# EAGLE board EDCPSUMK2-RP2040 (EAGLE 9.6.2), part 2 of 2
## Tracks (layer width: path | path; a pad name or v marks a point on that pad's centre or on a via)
1V1MCU  (via drill 0.3, 0.4)
  Top 0.203: U1.23 81.57,40.41 81.06,39.9 v81.06,39.74 | U1.45 88.21,39.21 87.54,39.88 87.54,41.22 v87.83,41.51 88.13,41.21 U1.50
  Bottom 0.203: C32.2 79.91,39.12 80.86,39.12 81.06,39.32 v81.06,39.74 82.73,39.74 83.25,39.22 87.47,39.22 87.5,39.25 | v87.83,41.51 87.54,41.22 87.54,39.29 87.5,39.25 | 87.5,39.25 87.5,38.11 C46.1 87.58,38.03 87.58,36.08 C33.2
3V3MCU  (via drill 0.3, 0.35, 0.4, 0.4 pad 0.9, 0.41 pad 0.81, 0.41 pad 0.91)
  Top 0.203: 39.17,32.42 39.17,34.39 C60.2 v40.17,36.38 | v80.92,40.6 81.13,40.81 U1.22 | R53.2 75.84,34.32 v75.19,34.32 | v91.78,36.41 91.29,36.91 91.29,38.01 90.49,38.81 U1.44 87.85,38.81 | U1.33 84.62,38.88 84.84,39.1 87.56,39.1 87.85,38.81 | 87.85,38.81 88.22,38.44 U1.42 88.22,35.7 89.01,34.91 C7.2 | U1.10 84.62,43.09 84.77,42.94 87.95,42.94 | 87.95,42.94 87.96,42.94 88.23,43.2 U1.1 | v87.96,43.38 87.96,42.95 87.95,42.94 | U1.49 88.26,40.81 88.1,40.65 v88.1,40.57 88.26,40.41 U1.48
  Top 0.305: J6.2 42.07,58.84 C25.2 | 41.83,52.58 C26.1 41.89,52.79 39.93,50.83 D3.2 | 2.28,36.83 R13.2 | U6.14 63.22,43.16 63.22,43.28 63.12,43.38 v62.4,43.38 65.71,46.69 C52.2 66.25,48.27 R15.1 | U3.14 70.06,40.65 69.92,40.51 v69.74,40.51 | U9.1 11.6,10.54 11.3,10.24 v11.02,10.24 v11.02,10.25 | R52.2 78.58,16 79.58,17.01 80.02,17.01 v80.3,17.29 | v14.29,19.85 14.29,21.84 K1.4 14.34,23.2 14.35,23.2 14.35,25.1 13.4,26.05 12.82,26.05 12.48,26.38 | 12.48,26.38 D7.2 | C57.1 9.45,25.95 10.12,25.95 | 10.12,25.95 12.05,25.95 12.48,26.38 | v10.07,26 10.12,25.95 | v46.01,40.72 47.28,41.99 48.53,41.99 LS1.1 | U2.3 39.01,32.26 39.17,32.42 | U5.8 78.31,57.28 v76.88,57.28
  Top 0.61: C25.2 41.83,52.58 | 2.28,36.83 C2.2 | R54.2 90.49,15.33 v89.82,16.01 | R35.1 58.67,49.62 58.32,49.28 v58.32,48.77 | R66.1 56.53,49.27 v56.29,49.03 | C44.2 28.08,33.71 v27.6,34.19 27.4,34.39 U7.1 | C7.2 90.9,34.91 C16.2 C45.1 92.37,35.78 | 92.39,35.8 92.37,35.78 | 92.37,35.78 92.37,35.83 v91.78,36.41
  Top 0.813: R13.2 1.63,36.87 v0.92,37.58
  PWR 0.305: v14.29,19.85 14.29,17.82 10.46,13.99 10.46,10.8 v11.02,10.25 | v0.92,37.58 0.92,35.51 | v10.07,26 8.75,26 8.04,26.71 8.04,28.91 7.83,29.12 3.6,29.12 2.59,30.13
  Bottom 0.203: v80.92,40.6 80.89,40.57 79.89,40.57 C50.2 | R40.2 78.17,55.88 v77.07,54.78
  Bottom 0.305: C20.2 61.25,43.06 62.08,43.06 v62.4,43.38 | v40.17,36.38 39.23,37.32 C51.2 | v91.78,36.41 91.8,36.41 92.55,35.66 R57.2 | 3V3MCU.TP 77.83,54.02 v77.07,54.78 | v76.88,57.28 78.66,59.06 81.7,59.06 C8.2 81.72,57.58 C15.1
  Bottom 0.61: D2.2 21.9,34.64 23.06,33.49 26.89,33.49 v27.6,34.19 | C53.2 v69.75,40.52 v69.74,40.51 | v89.82,16.01 89.86,16.05 89.86,18.4 90.5,19.04 90.5,21.93 90.36,22.07 | R19.2 90.36,22.07 | v87.96,43.38 87.45,43.89 | 87.45,43.89 C5.2 C6.2 | JP1.1 94.4,42.88 v94.4,43.49 | C31.2 87.45,43.89 | C12.2 88.01,25.69 88.01,24.45 88.69,23.77 89.41,23.77 90.5,22.68 90.5,22.21 90.36,22.07
  other vias: 72.48,54.67 73.17,55.87 74.11,56.29 73.17,56.91 73.13,57.69 73.1,58.55 74.09,57.38 75.07,54.8 76.81,56.25
  pour PWR (isolate 0.305, rank 3): -0.25,28.74 -0.25,53.44 7.21,60.9 91.95,60.9 97.18,55.67 97.18,7.88 74.15,7.88 74.15,50.26 70.2,50.26 70.2,36.19 35.77,35.9 32.88,32.99 11.08,33.28 11.08,49.14 4.17,49.14 3.97,28.74
  pour Top: 70.1,60.33 72.91,60.33 74.92,58.32 76.94,58.32 77.33,57.93 77.33,54.11 77.36,54.08 71.82,54.08 70.1,55.8
3V_REF  (via drill 0.35)
  Top 0.203: U1.43 90.25,38.41 90.77,37.89 90.77,37.04 89.59,35.86 v89.08,35.86
  Bottom 0.305: R57.1 89.62,32.35 89.39,32.12 | 89.39,32.12 89.39,29.32 90,28.71 C66.2 91.23,28.5 U8.1 | v89.08,35.86 89.06,35.86 89.06,32.45 89.39,32.12
BUZZ  (via drill 0.3)
  Top 0.203: U1.32 84.24,37.55 84.24,36.16 v84.29,36.11
  Bottom 0.305: R28.1 67.12,39.28 75.56,39.28 79.79,35.05 83.84,35.05 84.29,35.5 v84.29,36.11
CC1
  Bottom 0.305: J1.3 18.44,7.11 16.55,9 16.55,12.05 15.38,13.23 U10.13 10.91,13.23 9.51,14.62 7.82,14.62 R55.2
CC2
  Bottom 0.305: J1.9 15.45,7.65 15.45,11.85 14.72,12.57 U10.12 8.02,12.57 R56.2
CS
  Top 0.305: J6.7
  Top 0.61: J6.7 R29.2 R66.2
D0
  Top 0.305: J6.3
  Top 0.61: R14.2 J6.3
D1
  Top 0.305: J6.4
  Top 0.61: R17.2 J6.4
DSP_RST  (via drill 0.3, 0.3 pad 0.64)
  Top 0.203: U1.9 85.02,45.85 v84.19,46.68
  Top 0.305: R21.1 49.7,51.92 49.7,49.08 v49.68,49.05
  Bottom 0.203: v84.19,46.68 84.06,46.81 79.37,46.81 78.69,46.12 72.97,46.12 72.26,45.41 72.26,43.98 71.65,43.37 70.53,43.37 68.16,45.75 53.07,45.75 49.72,49.09 v49.68,49.05
EN_DCDC  (via drill 0.3, 0.3 pad 0.64)
  Top 0.203: U1.4 87.02,46.16 v87.42,46.56 v87.42,46.57
  Top 0.305: R31.1 61.57,48.57 v61.62,48.52
  Bottom 0.203: v87.42,46.57 86.32,46.57 85.14,47.76 78.74,47.76 78.04,47.06 69.84,47.06 69.42,47.48 62.93,47.48 62.43,46.98 60.09,46.98
  Bottom 0.305: v61.62,48.52 60.09,46.98 59.58,46.48 53.73,46.48 50.39,49.81 33.85,49.81 33.15,49.11 22.64,49.11 16.03,42.5 13.66,42.5 12.8,43.35 12.8,44.44 11.93,45.31 11.93,48.62 R27.2
EN_TPS54531  (via drill 0.3 pad 0.64)
  Top 0.305: U12.3 10.05,46.02 v9.8,46.28
  Bottom 0.305: 8.14,41.45 7.52,40.84 Q4.2 | v9.8,46.28 8.15,44.63 8.15,41.46 8.14,41.45 | 8.14,41.45 R43.2 6.08,39.76 5.41,39.09 EN_TPS54531.TP
FB
  Top 0.203: U11.1 70.05,47.99 70.28,47.76 FB_ADJ.2
FB_DAC
  Top 0.305: R30.1 36.7,34.16 U2.1
GND  (via drill 0.3, 0.3 pad 0.6, 0.3 pad 0.64, 0.35, 0.4, 0.4 pad 0.9, 0.41, 0.41 pad 0.81, 0.41 pad 0.91, 1.5 pad 2.5)
  Top 0.203: U1.19 84.17,42.01 v84.4,42.24 | 90.9,33.11 C16.1 | U2.2 v37.9,33.01 | U1.57 85.61,41.02 v85.61,41.08 | U12.9 14,46.76 v14,46.99
  Top 0.305: 19.33,47.4 C38.1 | U6.7 57.42,38.73 v56.79,38.1 | U7.9 18.31,30.65 v17.7,30.65 17.22,30.65 R50.2 14.63,33.24 C58.1 | Q5.2 5.52,15.93 R49.1 6.7,19.02 v8.32,20.65 8.32,21.72 C57.2 | C54.1 69.61,45.09 v70.84,45.09 | v62.74,34.65 64.45,34.65 65.56,33.54 C48.1 | C2.1 4.18,34.68 6.75,34.68 v6.76,34.67 6.55,34.67 5.87,35.36 S2.2 | v12.31,30.27 12.81,29.77 D7.1 | v41.99,36.48 41.99,35.41 C60.1 41.97,34.64 41.5,34.17 U2.6 | R16.2 64.66,50.11 Q2.2 | v74.19,59.83 74.46,59.56 DZ1.2 76.18,59.56 v76.41,59.79 | 1.93,41.78 1.71,41.56 | U12.7 15.47,47.3 v15.01,47.76 | C65.1 32.34,31.61 32.99,31.61 v33.06,31.68 33.8,31.68 R45.1 | C27.1 49.92,33.48 v50.25,33.81 | U3.7 73.95,37.35 75.04,38.44 C61.1 75.24,38.47 75.24,39.95 75.55,40.26 X1.2 76.2,40.31 v76.2,41.68 | U4.2 U4.1 39.02,39.88 v38.49,39.35 | 78.67,45.16 78.67,44.17 X1.4 | 78.67,45.16 C59.1 | U5.4 83.45,50.3 v83.48,50.27 | v79,45.49 78.67,45.16 | C16.1 91.64,32.37 v91.64,31.15
  Top 0.508: 1.68,45.79 1.71,45.76 C21.2 1.64,44.67 0.57,44.67 | 4.62,45.6 4.6,45.58 C17.2 4.6,43.79 | C18.2 7.55,44.52 7.55,45.65 | 4.6,43.79 | C18.2 7.56,43.76 7.54,43.74 | C18.2 7.57,44.52 8.82,44.52
  Top 0.61: 19.33,47.4 19.33,47.88 19.64,48.19 R44.1 19.64,50.44 v19.7,50.51 | v23.55,45.35 22.84,44.64 C34.1 | v95.02,16.06 94.44,16.65 C24.1 | U7.9 U7.10 | v18.44,34.17 18.51,34.23 U7.8 U7.7 | C44.1 27.77,31.91 27.66,31.8 v27.46,31.8 27.4,31.74 U7.16 | C26.2 40.03,52.79 C25.1 40.03,55.94 J6.1 | C11.1 55.19,37.86 56.55,37.86 v56.79,38.1 | C49.1 67.05,40.76 66.49,40.2 v66.38,40.2 | C47.1 v70.84,45.09 | v54.38,47.25 54.94,47.25 C9.2 | Q2.2 64.63,48.85 v64.62,48.82 | R18.1 59.65,42.36 v59.33,42.04 | 85.46,9.49 v85.3,9.33 | v62.74,34.65 62.7,34.69 C14.1 | 18.35,23.28 K1.9 18.35,22.12 18.46,22.23 v19.04,22.23 | 18.35,23.28 18.35,23.51 18.33,23.51 18.33,26.67 v18.3,26.71 17.35,25.75 K1.8 | C45.2 C16.1 90.9,33.11 | C16.1 89.47,33.09 C7.1 | v19.29,23.28 18.35,23.28 | v19.3,21.02 18.41,21.02 18.35,20.96
  Top 0.813: C21.2 1.71,41.56 v0.79,40.64 | OP1.3 85.46,9.49 | C10.1 1.93,41.78 | v19.55,15.3 19.81,15.04 RSENSE.2
  Top 1.016: R59.1 17.6,15.3 v19.55,15.3 | D6.1 13,54.63 | D6.1 15.33,51.7 | D6.1 15.33,57.6 | D6.1 15.65,54.3 17.15,54.3
  Top 1.27: C21.2 4.57,44.6 C17.2 7.44,44.63 C18.2
  Bottom 0.203: 85.45,45.64 86.76,45.64 C5.1 v87.62,45.71 C31.1
  Bottom 0.305: v18.44,34.17 18.92,34.64 D2.1 | v12.31,30.27 12.31,29.05 C35.2 | C36.1 6.76,32.67 v6.76,34.67 | D8.2 14.46,39.94 12.69,41.71 v9.04,41.71 | C28.1 5.95,45.19 5.95,44.68 6.28,44.35 6.28,44.05 6.4,44.05 v6.5,43.95 | v9.04,41.71 9.16,41.83 9.16,43.67 C30.1 | R43.1 9.94,40.81 v9.04,41.71 | C15.2 83.55,59.05 C8.1 v84.58,59.08 v84.59,59.09 | C51.1 37.86,34.42 37.91,34.37 v37.91,33.02 v37.9,33.01 | C12.1 89.98,25.83 | Q9.2 60.86,35.83 R32.2 62.05,35.34 v62.74,34.65 | C32.1 78.11,39.16 C50.1 77.29,40.59 v76.2,41.68 | C42.2 23.71,45.51 v23.55,45.35 | U8.2 92.7,30.51 C66.1 91.64,31.13 v91.64,31.15 | GND.TP 40.42,58.5 39.53,57.61 J6.1
  Bottom 0.61: 31.69,45.59 C39.2 31.63,45.53 35.91,45.53 36.2,45.81 v36.2,46.66 | C53.1 72.55,40.21 72.72,40.04 v72.81,40.04 | C22.1 82.82,20.19 v82.96,20.32 | C23.1 80.66,23.49 v80.55,23.37 | C20.1 60.11,41.27 v59.33,42.04 | S1.SW- 89.98,25.66 89.98,25.83 | C6.1 85.45,45.64 | 86.58,45.64 86.78,45.66 C5.1 | JP1.3 JP1.5 JP1.7 JP1.9 94.02,36.21 v94.06,36.17 | C46.2 85.83,37.98 C33.1 85.19,36.03 v85.12,36.09
  Bottom 0.813: C42.2 C40.2 28.61,45.56 31.56,45.56 C39.2 | R22.2 82.28,12.17 v82.66,11.79
  Bottom 1.016: v20.92,22.07 20.92,23.74 20.5,24.16
  other vias: 13.54,53.09 14.25,47.76 13.49,47.76 13.23,46.99 14.76,46.99 15.01,46.23 14.25,46.23 13.49,46.23 13.23,45.47 14,45.47 14.76,45.47 14.27,50.96 14.77,51.96 15.27,50.96 16.27,50.96 15.77,51.96 16.77,51.96 17.27,50.96 17.77,51.96 17.27,52.96 13.77,51.96 9.77,56.46 10.77,56.46 11.77,56.46 12.77,56.46 20.77,50.96 13.77,56.46 21.77,50.96 22.77,50.96 11.32,59.76 12.32,59.76 13.32,59.76 14.32,59.76 15.32,59.76 16.32,59.76 17.32,59.76 18.32,59.76 19.32,59.76 20.32,59.76 21.32,59.76 22.32,59.76 23.32,59.76 24.32,59.76 25.32,59.76 26.32,59.76 27.32,59.76 15.82,50.26 10.82,58.76 11.82,58.76 12.82,58.76 13.82,58.76 14.82,58.76 15.82,58.76 16.82,58.76 17.82,58.76 18.82,58.76 19.82,58.76 20.82,58.76 21.82,58.76 22.82,58.76 23.82,58.76 24.82,58.76 25.82,58.76 26.82,58.76 14.82,50.26 11.32,57.76 12.32,57.76 13.32,57.76 14.32,57.76 15.32,57.76 16.32,57.76 17.32,57.76 18.32,57.76 19.32,57.76 20.32,57.76 21.32,57.76 22.32,57.76 23.32,57.76 24.32,57.76 25.32,57.76 26.32,57.76 9.4,55.3 10.4,55.3 11.4,55.3 12.4,55.3 9.9,54.3 10.9,54.3 11.9,54.3 12.9,54.3 9.4,53.3 10.4,53.3 11.4,53.3 12.4,53.3 9.9,52.3 10.9,52.3 11.9,52.3 12.9,52.3 28.97,51.23 29.99,51.23 31.11,51.27 32.21,51.31 6.5,44.69 18.95,16.5 20.55,16.49 20.92,15.25 72.96,52.92 72.95,51.91 74.2,52.18 75.15,52.17 76.28,52.17 77.14,52.9 77.2,51.7 85.6,42.24 86.81,42.24 86.81,41.08 86.81,39.92 85.6,39.92 84.4,39.92 84.4,41.08 18.27,25.73 19.31,24.43
  pour Bottom: 11.94,49.38 11.94,45.32 12.8,44.45 12.8,43.18 13.57,42.42 15.88,42.42 18.34,44.89 18.34,47.96 18.75,48.37 18.75,49.08 18.44,49.38
  pour Top (no thermals): 85.96,10.47 85.96,8.44 89.77,8.44 89.77,10.47
  pour Top: 8.9,60.3 8.9,52.32 11.42,49.8 33.4,49.8 32.9,50.3 32.9,59.8 32.4,60.3
  pour Bottom (isolate 0.305): 8.41,60.3 8.41,48.79 12.9,44.3 18.4,44.3 22.9,48.8 32.9,48.8 33.4,49.3 33.4,59.8 32.9,60.3
  pour GND (isolate 0.35): -1.04,13.55 24.58,13.55 24.58,27.1 74.2,27.1 74.2,5 97.89,5 97.89,54.02 89.91,62 6.05,62 -1.04,54.91
  pour Top: 18.29,14.04 21.73,14.04 21.73,17.59 18.29,17.59
  pour Top: 0.25,46.26 0.25,43.56 9.22,43.56 9.22,46.34 0.25,46.34 0.25,46.27
  pour Bottom (isolate 0.254): 17.09,28.7 18.78,28.7 18.78,23.84 22.21,23.84 22.21,20.52 16.99,20.52 16.99,28.51
  pour Top: 71.68,53.57 77.4,53.57 77.4,51.38 76.87,50.85 73.36,50.85 72.37,51.84 71.68,51.84
  pour Bottom: 23.44,47.1 36.78,47.1 36.78,44.88 36.48,44.58 22.71,44.58 22.71,46.37
  pour Bottom (isolate 0.254): 22.39,20.57 22.39,28.01 41.36,28.01 41.36,32.72 40.92,33.16 17.77,33.16 16.91,32.3 16.91,20.51
  pour Top (isolate 0.254): 17.4,27.46 19.13,27.46 19.82,26.77 19.82,24.1 20.12,23.8 21.93,23.8 22.39,23.34 22.39,21.33 21.63,20.57 18.98,20.57 18.89,20.66 18.89,23.76 18.39,24.26 17.14,24.26 17.02,24.38 17.02,27.08
GND_IN  (via drill 0.3 pad 0.6, 0.3 pad 0.64, 0.4 pad 0.8)
  Top 0.203: J1.S5 20.19,1.12 D4.3 13.21,1.12 J1.S6
  Top 0.305: R34.1 10.2,16.2 v9.85,16.55 | U9.3 13.55,11.09 13.55,9.45 13.27,9.73 12.55,9.73 U9.2 U9.3
  Top 1.016: C56.2 16.78,7.99 16.78,8.16 16.84,8.11 16.84,9.55 16.63,9.75 C55.2 16.75,11.01 19.56,11.01 RSENSE.1 19.81,8.9 v20.04,8.67
  Bottom 0.203: 6.15,15.55 6.1,15.5 R55.1 5.3,14.6
  Bottom 0.305: 5.3,14.6 4.56,13.86 v4.56,12.68 4.58,12.66 6.09,12.66 R56.1 | J1.12 v13.59,7.62 | J1.1 19.8,7.12 v20.09,7.42 | U10.5 18.11,12.56 18.99,12.56 20.04,11.51 v20.04,8.67 | 6.15,15.55 7.33,16.73 9.67,16.73 v9.85,16.55 5.55,16.55 GND_IN.TP
  other vias: 21.29,8.62 21.29,7.47 12.39,8.67 13.59,8.67 12.44,7.62
  pour GND: -1.3,12.8 24.2,12.8 24.2,-2 -1.3,-2
  pour Top: 7.26,6.8 21.7,6.8 21.7,11.55 7.26,11.55
  pour Bottom (isolate 0.254): 19.4,9.22 22,9.22 22,0.35 11.4,0.35 11.37,0.38 11.37,9.12 11.45,9.2 14.2,9.2 14.2,6.9 13.65,6.9 13.65,2.9 19.5,2.9 19.85,3.25 19.85,5.35 19.4,5.8
IN+  (via drill 0.3 pad 0.6, 0.3 pad 0.64, 0.35, 1.5 pad 2.5)
  Top 0.203: PTC1.2 2.84,29.71
  Top 0.305: 3.32,11.45 3.04,11.73 v2.99,11.73
  Top 0.406: D1.C 2.52,10.18 2.4,10.3
  Top 1.016: C56.1 16.8,6.11 | 16.78,5.03 16.78,6.15 C56.1 | C56.1 16.92,6.05 | v6.4,27.09 5.47,27.09 2.84,29.71
  Bottom 0.305: J1.2 19.05,5.54 18.45,4.94 v18.44,4.94 | R47.1 v21.39,11.05 | v15.03,4.86 14.35,5.54 J1.11 | R62.2 6.07,10.52 4.2,10.52 v2.99,11.73 2.02,12.7 IN+.TP
  Bottom 0.61: R51.1 6.02,36.41 5.08,35.47 C36.2 5.08,30.37 6.43,29.02 6.43,27.12 v6.4,27.09
  other vias: 14.44,3.97 19.06,3.85 16.8,3.9 2.95,10.99 3,9.58
  pour Bottom (isolate 0.254, rank 2): 13.89,5.89 13.89,3.26 19.79,3.26 19.79,5.89
  pour Top: 13.77,6.06 19.79,6.06 19.79,3.29 13.77,3.29
  pour PWR (isolate 0.254): -0.6,28.87 -0.6,10.35 11.05,-1.3 23.9,-1.3 23.9,17.7 23.8,17.8 7.88,17.8 7.88,28.87
  pour Top (isolate 0.305): 2.61,11.99 2.16,11.54 2.16,9.11 3.34,7.93 4.16,7.93 4.46,8.23 4.46,11.59 4.05,12 2.63,12
IN_OVC  (via drill 0.3, 0.35)
  Top 0.305: R48.2 6.7,12.69 R49.2 | R49.2 6.57,14.11 Q5.1 | v12.66,25.19 11,25.19 10.15,24.34 10.15,18.98 8.12,16.95 8.12,14.67 7.63,14.18 R49.2 | v66.46,32.13 66.5,32.17 66.5,39.17 67.21,39.88 68.87,39.88 68.92,39.93 68.92,41.51 69.42,42 70.42,42 70.6,42.18 70.6,43.62 70.35,43.87 64.55,43.87 64.27,43.59 64.27,42.6 64.12,42.45 U6.13
  GND 0.305: v37.06,31.59 36.42,30.94 18.7,30.94 18.25,31.39 16.89,31.39 16.23,30.73 v16.23,30.01
  PWR 0.305: v66.46,32.13 66.3,31.97 40.08,31.97 39.74,32.31 38.98,32.31 38.26,31.59 v37.06,31.59 | v16.23,30.01 15.44,30.01 12.66,27.23 v12.66,25.19
ISENSE  (via drill 0.3, 0.4)
  Top 0.203: U1.39 87.04,37.55 87.04,33.97 86.81,33.74 v86.81,33.59
  Top 0.305: U4.3 41.06,40.84 v40.89,41.02
  Bottom 0.305: v86.81,33.59 86.71,33.49 78.4,33.49 76.16,35.73 73.99,35.73 71.91,37.81 69.11,37.81 65.06,33.76 59.22,33.76 57.57,35.41 45.12,35.41 40.89,39.64 v40.89,41.02 40.47,41.44 ISENSE.TP
MISO  (via drill 0.3, 0.3 pad 0.64)
  Top 0.203: v81.45,36.96 81.23,37.18 81.23,38.49 81.55,38.81 U1.27
  Top 0.305: R24.1 53.12,51.94 v53.49,51.57
  PWR 0.203: v81.45,36.96 81.23,37.18 81.23,37.94 81.46,38.17 87.48,38.17 88.74,39.43 88.74,47.28 88.2,47.82 v87.92,47.82
  Bottom 0.305: v53.49,51.57 53.64,51.42 70.71,51.42 71.57,50.56 82.84,50.56 83.21,50.93 84.26,50.93 87.37,47.82 v87.92,47.82
MOSI  (via drill 0.3, 0.3 pad 0.64)
  Top 0.203: U1.30 83.44,37.55 v83.44,36.25 v83.43,36.24
  Top 0.305: R17.1 48.3,51.94 v48.41,51.82
  PWR 0.203: v83.43,36.24 83.43,36.73 88.33,36.73 90.15,38.56 90.15,47.85 87.3,50.7 v85.37,50.7
  Bottom 0.203: v85.37,50.7 84.63,51.44 84.52,51.44
  Bottom 0.305: v48.41,51.82 50.16,53.57 69.58,53.57 72.06,51.09 77.45,51.09 77.8,51.44 84.52,51.44
N$1
  Top 0.305: U7.6 21.05,36.9 21.72,37.57 R3.1
N$2
  Top 0.305: U7.5 22.32,36.29 23.49,37.47 R4.1
N$3
  Top 0.305: U7.4 23.59,36.39 25.15,37.95 25.17,37.95 R5.1
N$4
  Top 0.305: U7.3 24.86,36.34 25.65,37.13 26.13,37.13 R6.1
N$5  (via drill 0.3 pad 0.64)
  Top 0.305: R7.1 30.61,37.88 v31.4,37.09 | U7.14 24.86,31.64 v24.84,31.64
  Bottom 0.305: v31.4,37.09 29.62,35.31 29.62,32.39 28.14,30.91 26.89,30.91 26.16,31.64 v24.84,31.64
N$6
  Top 0.305: J6.6
  Top 0.61: R24.2 J6.6
N$7  (via drill 0.3 pad 0.64)
  Top 0.305: R8.1 28.83,37.37 v29.11,37.09 | U7.13 23.56,30.46 v23.56,31.63
  Bottom 0.305: v29.11,37.09 28.91,36.89 28.91,33.43 28.17,32.69 23.56,32.69 v23.56,31.63
N$8
  Top 0.305: U7.12 22.32,32.2 21.34,33.18 18.03,33.18 17.43,33.79 17.43,36.63 17.93,37.13 19.79,37.13 R9.1
N$9
  Top 0.305: U7.11 21.05,32.1 20.73,32.42 17.58,32.42 16.7,33.3 16.7,34.1 16.21,34.59 13.06,34.59 12.6,35.06 12.6,37.09 13.36,37.85 17.74,37.85 R10.1
N$10
  Top 0.305: C43.2 41.06,45.37 U4.4 41.79,42.42 42.18,42.03 42.18,37.86 R1.1
N$11
  Top 0.61: R35.2 59.55,52.29 61.88,54.61 61.88,55.29 LED1.A
N$12
  Top 0.61: Q2.3 63.98,54.86 LED1.K
N$13
  Top 0.305: R33.1 62.57,37.67 60.35,37.67 58.17,39.85 U6.6
N$14
  Bottom 0.305: R62.1 9.15,10.7 10.38,11.93 U10.11
N$15
  Top 0.305: U6.12 64.35,41.8 64.72,42.17 65.18,42.17 65.51,42.5 R39.1
N$16  (via drill 0.3)
  Top 0.305: v56.82,33.27 56.82,31.45 D5.2 | v76.99,12.07 79.78,12.07 OP1.1
  Bottom 0.305: v56.82,33.27 60.09,30 75.62,30 76.79,28.83 76.79,12.27 v76.99,12.07
  pour Top (no thermals): 77.58,13.01 77.58,10.98 80.88,10.98 80.88,13.01
N$17
  Top 0.305: 6,39.98 S2.4 6.25,40.49
  Top 0.61: R13.1 5.55,38.67 6,39.12 6,39.98 | C10.2 5.89,41.76 6.25,41.41 6.25,40.49 | S2.4 10.54,40.1 12.49,42.05 R65.2
N$18
  Top 0.305: U3.9 73.31,42.68 74.08,43.45 R2.2 74.25,44.94 C47.2
N$19
  Top 0.305: 19.35,42.5 C19.1 19.27,42.42 18.7,42.42 17.93,41.66 R10.2 R9.2 21.7,39.84 R3.2 R4.2 R5.2 R6.2 R8.2 R7.2 32.2,38.25 32.2,33.49 C65.2 R45.2 33.92,33.36 34.45,33.36 34.82,32.99 34.82,32.3 35.52,31.61 R30.2 | R11.1 18.67,44.02 17.94,44.76 U12.5
  Top 0.61: R11.1 19.35,42.5
N$20
  Bottom 0.305: Q9.1 59.84,37.14 R32.1 62.76,37.14 R28.2
N$21
  Top 0.61: R31.2 62.59,51.36 63.33,50.62 Q2.1
N$22
  Top 0.305: U3.10 72.65,41.16 72.65,43.25 R2.1
N$23
  Top 0.305: U3.6 73.31,33.39 R20.1
N$25
  Top 0.305: U3.2 70.7,36.48 69.49,36.48 68.83,35.82 R25.1
N$26
  Top 0.305: R25.2 67.82,37.89 C49.2 67.98,39.12 70.7,39.12 U3.13
N$28
  Top 0.305: U3.3 71.36,33.58 71.43,33.5 R20.2 71.43,32.27 70.89,31.73 68.08,31.73 67.36,32.45 C48.2
N$29
  Top 0.305: C11.2 R23.2 55.16,41.55 55.41,41.8 U6.3
N$31  (via drill 0.3)
  Top 0.203: BZ1.2 48.64,46.6 LS1.2
  Top 0.305: BZ1.2 43.67,46.7 42.04,48.33 D3.3 | LS1.2 49.59,46.51 52.17,43.93 52.17,37.91 53.81,36.27 56.83,36.27 v57,36.1 56.84,36.26 53.85,36.26 52.89,35.3 R61.1
  Bottom 0.305: Q9.3 57.38,36.48 v57,36.1
N$32  (via drill 0.41 pad 0.81)
  Top 0.305: 47.3,36.35 BZ1.1 | L7.2 49.14,35.3 C27.2 50.81,35.28 R61.2
  Top 0.61: L7.2 47.3,36.35 | v47.45,39.73 48.64,38.54 BZ1.1
N$34
  Top 0.305: U6.2 56.2,42.45 55.98,42.68 55.22,42.68 R23.1
N$35
  Bottom 0.305: R41.1 3.9,41.49 Q4.3
N$37
  Top 0.305: U6.9 64.09,39.85 64.44,39.5 R33.2 64.44,36.12 C14.2
N$38
  Top 0.203: R16.1 R15.2 | R15.2 67.98,46.76 C52.1 | FB_ADJ.1 69.27,46.77 69.25,46.79 67.98,46.79 R15.2
N$39
  Top 0.305: R39.2 65.94,41.15 67.81,43.03 C54.2 | U6.11 R39.2 | R39.2
N$40  (via drill 0.3 pad 0.64)
  Top 0.305: U7.2 26.12,34.45 v26.12,34.44 | L6.1 28.97,36.16 v28.09,37.03
  Bottom 0.305: v28.09,37.03 26.52,37.03 25.81,36.33 25.81,34.75 v26.12,34.44
N$41  (via drill 0.41 pad 0.91)
  Top 0.305: 81.72,9.49 v81.95,9.71
  Top 0.813: OP1.2 81.72,9.49
  Bottom 0.305: R26.2 80.99,9.71 v81.95,9.71 83.76,9.71 85.02,10.97 N$41.TP
  pour Top (no thermals): 77.64,10.47 77.64,8.44 80.88,8.44 80.88,10.47
N$43  (via drill 0.35)
  Top 0.203: L3.2 74.18,29.21 v74.3,29.09
  Bottom 0.203: v74.3,29.09 75.81,29.09 76.28,28.62 76.28,11.29 77.89,9.68 R26.1
N$44  (via drill 0.3 pad 0.64)
  Top 0.305: v11.84,43.69 11.41,44.12 11.41,44.74 U12.4
  Bottom 0.305: C30.2 v11.84,43.69
N$45
  Top 0.305: U2.5 43.79,33.21 44.21,32.79 R58.2
N$46  (via drill 0.3 pad 0.64)
  Top 0.305: L4.2 v78.92,13.76
  Bottom 0.305: v78.92,13.76 78.94,13.73 R22.1
N$47
  Top 0.61: C29.1 11.13,49.57 11.4,49.3 U12.1
N$48
  Top 0.305: U2.4 42.15,32.26 R60.2
N$50
  Bottom 0.305: R47.2 20.8,14.52 U10.2
N$51  (via drill 0.35)
  Top 0.305: L2.1 30.82,54.47 v31.29,54.95
  Top 0.61: U12.8 16.8,49.23 16.75,49.28 | 16.75,49.28 17.16,49.28 18.68,50.8 18.68,53.33 19.97,54.62 D6.2 | 16.75,49.28 13.36,49.28 12.93,49.71 C29.2
  Top 1.016: D6.2 22.9,53.25 28.77,53.25 L2.1
  Bottom 0.305: v31.29,54.95 31.29,57.35 N$51.TP
N$52
  Top 0.61: C37.2 C38.2 18.9,46.02 U12.6
N$53
  Top 0.61: R44.2 21.44,47.2 C37.1
N$54
  Top 0.305: U7.15 26.12,29.18 27.9,29.18 28.43,29.71 L5.1
N$56
  Top 0.305: U11.6 70.02,53.13 C4.2
N$58
  Top 0.305: U9.5 11.6,12.77 11.51,12.68 R48.1
N$59  (via drill 0.35)
  Top 0.305: C55.1 15.79,13.86 U9.4 13.5,14.84 13.94,15.29 R59.2 | R34.2 13.95,16.2 14.86,15.29 R59.2 | v15.6,16.86 15.6,15.52 R59.2
  Bottom 0.305: v15.6,16.86 15.13,16.86 N$59.TP
N$63
  Top 0.203: C61.2 78.26,38.44 78.21,38.49 78.17,38.49
  Top 0.305: X1.3 78.17,39.88 78.17,38.49 R46.2
N$64  (via drill 0.3, 0.4)
  Top 0.305: USB_D+.1 21.89,28.21 v21.6,28.5 | v81.83,31.48 81.99,31.32 81.99,27.93 83.71,26.21 90.17,26.21 95.48,31.52 95.48,39.83 94.75,40.56 R38.1
  PWR 0.305: v21.6,28.5 21.6,28.68 22.54,29.62 34.86,29.62 36.14,30.91 81.14,30.91 81.71,31.48 v81.83,31.48
N$65  (via drill 0.3, 0.4)
  Top 0.203: R63.1 94.78,38.94
  Top 0.305: v21.9,24.75 21.88,24.77 USB_D-.1 | v82.82,30.74 82.82,28.15 83.91,27.05 89.67,27.05 94.78,32.17 94.78,38.94
  PWR 0.305: v21.9,24.75 22.29,24.75 22.29,28.57 22.79,29.07 35.12,29.07 36.44,30.39 82.47,30.39 v82.82,30.74
N$67
  Top 0.305: 68.4,54.91 C4.1
  Top 0.61: U11.5 71,54.13 70.22,54.91 68.4,54.91
  Top 0.813: L1.1 68.47,54.93 C4.1
  pour Top: 69.06,60.43 69.06,54.22 69.08,54.2 66.64,54.2 66.61,54.23 66.61,60.38 66.71,60.48 68.86,60.48
OVC_ALARM  (via drill 0.3, 0.41 pad 0.81)
  Top 0.203: U1.12 83.82,43.78 v84.06,43.54
  Top 0.305: U6.10 64.26,40.5 65.45,39.32 65.55,39.18 v65.55,39.06
  Bottom 0.203: 83.59,43.86 83.74,43.86 v84.06,43.54
  Bottom 0.305: v65.55,39.06 65.55,41.11 66.2,41.76 72.26,41.76 74.36,43.86 83.59,43.86 | OVC_ALARM.TP 82.5,45.1 v84.06,43.54
PDL  (via drill 0.35)
  Top 0.305: U6.1 56.76,43.1 56.47,43.5 56.47,44.75 56.28,44.94 C9.1 | R18.2 57.03,45.58 56.35,44.91 55.48,44.91 C9.1 | C9.1 53.94,44.94 53.38,44.38 53.38,37.56 53.97,36.97 59.01,36.97 65.03,30.95 75.84,30.95 v77.24,29.55
  PWR 0.305: v77.24,29.55 81.74,25.05 86.07,25.05 86.25,24.87 v86.72,24.87
  Bottom 0.61: R99.2 87.09,22.09 87.09,24.5 v86.72,24.87
PEDAL  (via drill 0.41 pad 0.91)
  Top 0.813: OP1.4 87.27,13.51 v88.6,14.84
  Bottom 0.305: R19.1 88.8,15.04 v88.6,14.84
  Bottom 0.61: R19.1 88.77,20.25 | 88.77,20.25 | 88.77,20.25 R99.1
  pour Top (no thermals): 85.96,13.01 85.96,10.98 89.77,10.98 89.77,13.01
PEDAL+  (via drill 0.3)
  Top 0.203: L3.1 71.57,29.79 v70.86,29.08
  Top 0.61: K1.2 12.34,19.57 12.37,19.55 v12.37,19.47
  GND 0.305: v12.37,19.47 13.92,21.02 16.97,21.02 17.48,21.53 17.48,27.05 18.53,28.1 20.1,28.1 21.19,29.2 36.28,29.2 v36.28,29.13
  PWR 0.305: v70.86,29.08 70.82,29.04 36.37,29.04 v36.28,29.13
  Bottom 0.305: v70.86,29.08 58.51,29.08 PEDAL+.TP
PEDAL-  (via drill 0.3)
  Top 0.305: 79.55,15.56 v78.87,14.88
  Top 0.61: L4.1 79.55,15.56 | v11.35,19.48 K1.1
  GND 0.305: v11.35,19.48 11.35,19.95 13.04,21.65 16.54,21.65 16.86,21.98 16.86,27.26 19.43,29.81 37.81,29.81 v37.91,29.73
  PWR 0.305: v78.87,14.88 76.39,17.35 76.39,28.79 75.39,29.79 37.97,29.79 v37.91,29.73
  Bottom 0.305: PEDAL-.TP 80.76,14.88 v78.87,14.88
PEDAL_IP  (via drill 0.3, 0.3 pad 0.64)
  Top 0.203: U1.11 84.22,45.87 83.95,46.14 v81,46.14
  Top 0.305: U6.4 59.33,41.15 v60.35,40.14
  Bottom 0.203: 78.77,44.86 79.22,44.86 80.5,46.14 v81,46.14
  Bottom 0.305: 78.77,44.86 74.23,44.86 71.88,42.51 64.75,42.51 62.58,40.34 60.55,40.34 v60.35,40.14
PUSH  (via drill 0.3 pad 0.64, 0.41 pad 0.81)
  Top 0.305: U6.5 58.71,40.5 v58.83,40.39
  Top 0.61: R65.1 17.06,42.05 v17.43,42.42
  Bottom 0.305: v17.43,42.42 23.03,48.02 38.72,48.02 44.12,42.62 56.6,42.62 v58.83,40.39
PUSH_FILT  (via drill 0.3, 0.3 pad 0.64)
  Top 0.203: U1.5 86.62,46.98 v86.88,47.24
  Top 0.305: U6.8 61.69,39.2 61.16,39.73 61.16,45.52 61.88,46.23 v61.88,47.6
  Bottom 0.203: v86.88,47.24 86.22,47.24 85,48.47 82.48,48.47 81.92,49.03 79.44,49.03 78.27,47.86 77.36,47.86 77.03,48.19 77.03,48.67 76.65,49.05 74.9,49.05 73.31,47.46 70.01,47.46 69.59,47.89 62.16,47.89 v61.88,47.6
QSPI_SCLK
  Top 0.203: U1.52 91.69,42.01 92.3,42.62 92.3,46.49 88.89,49.9 87.56,49.9 82.19,55.27 U5.6
QSPI_SD0  (via drill 0.3)
  Top 0.203: U1.53 91.06,42.41 91.71,43.06 v91.71,43.85 | v84.97,56.31 84,56.31 83.45,56.86 U5.5
  Bottom 0.203: v91.71,43.85 91.71,46.92 92.62,47.83 92.62,49.34 92.23,49.73 88.21,49.73 84.96,52.98 v84.96,56.3 v84.97,56.31
QSPI_SD1
  Top 0.203: U1.55 90.27,43.21 90.71,43.65 90.71,46.66 88.47,48.9 81.67,48.9 80.92,49.66 U5.2
QSPI_SD2
  Top 0.203: U1.54 90.52,42.81 91.13,43.42 91.13,46.97 88.69,49.41 82.6,49.41 82.19,49.83 U5.3
QSPI_SD3
  Top 0.203: U1.51 92,41.61 92.79,42.4 92.79,46.67 89.16,50.3 88.07,50.3 85.93,52.44 85.93,59.3 85.19,60.04 81.1,60.04 80.92,59.86 U5.7
QSPI_SS  (via drill 0.4)
  Top 0.203: U1.56 89.98,43.61 90.22,43.85 90.22,46.47 88.2,48.49 80.05,48.49 79.64,48.9 U5.1 v79.64,53.52
  Bottom 0.203: R40.1 83.53,54.47 82.58,53.52 v79.64,53.52
ROTA
  Top 0.305: U3.5 72.66,34.43 72.37,34.14 72.37,32.47 72.82,32.02 76.16,32.02 R53.1
  Top 0.813: R53.1 77.35,32.11 78.42,31.37 S1.A
  Bottom 0.813: C23.2 78.78,25.29
  Bottom 1.016: 78.78,25.29 S1.A
ROTA_FILT  (via drill 0.3, 0.41 pad 0.81)
  Top 0.203: v85.01,35.21 85.84,36.04 85.84,37.55 U1.36
  Top 0.305: v73.4,38.48 73.29,38.37 73.29,37.25 72.01,35.97 U3.4
  Bottom 0.305: v73.4,38.48 73.43,38.48 74.81,37.1 76.5,37.1 79.07,34.53 84.34,34.53 v85.01,35.2 v85.01,35.21
ROTB  (via drill 0.3 pad 0.64)
  Top 0.305: U3.11 72.03,41.15 72.03,37.07 v71.48,36.53
  Top 0.61: v85.4,21.94 79.76,21.94 77.81,19.99 R52.1 77.81,19.97 S1.B
  Top 0.813: S1.B
  Bottom 0.61: v71.48,36.53 71.48,33.86 72.15,33.19 76.57,33.19 85.54,24.22 85.54,22.07 v85.4,21.94
  Bottom 0.813: C22.2 79.81,21.99 S1.B
ROTB_FILT  (via drill 0.3, 0.4)
  Top 0.203: U1.15 80.23,43.61 v79.76,43.14
  Top 0.305: U3.8 73.95,41.94 74.31,42.29 74.92,41.67 v74.92,41.63
  Bottom 0.203: v79.76,43.14 79.57,42.95 78.9,42.95
  Bottom 0.305: v74.92,41.63 74.92,42.63 75.24,42.95 78.9,42.95
ROTPUSH  (via drill 0.3 pad 0.64)
  Top 0.305: U3.1 70.06,33.43 | S1.SW+ 92.89,15.85 92.63,15.58 R54.1
  Top 0.61: v81.09,26.87 84.14,23.82 89.65,23.82 S1.SW+ | 70.06,33.43 69.95,33.33 v69.95,32.82
  Top 1.016: C24.2 94.44,19.03 S1.SW+
  Bottom 0.61: v69.95,32.82 70.51,32.26 75.94,32.26 81.09,27.12 v81.09,26.87
RPUSH_FILT  (via drill 0.3, 0.3 pad 0.64)
  Top 0.203: U1.8 85.42,46.51 v85.15,46.78
  Top 0.305: v71.37,44 71.37,41.16 U3.12
  Bottom 0.203: 78.42,46.58 79.09,47.24 84.69,47.24 v85.15,46.78
  Bottom 0.305: 78.42,46.58 71.89,46.58 71.63,46.33 71.63,44.73 71.37,44.47 v71.37,44
RST
  Top 0.305: J6.5
  Top 0.61: R21.2 J6.5
RUN  (via drill 0.35)
  Top 0.203: U1.26 81.34,39.21 80.82,38.69 80.82,36.82 v80.62,36.62
  PWR 0.203: v80.62,36.62 82.03,35.21 84.09,35.21 84.74,34.56 85.55,34.56 87.05,36.06 88.26,36.06 89.66,37.46 v92.15,37.46
  Bottom 0.203: v92.15,37.46 92.11,37.42 JP1.10
  Bottom 0.305: v92.15,37.46 92.15,37 93.22,35.93 93.22,34.06 RUN.TP
SAFETY_EN_DCDC  (via drill 0.35)
  Top 0.305: v1.8,14.75 Q5.3
  Bottom 0.305: v1.8,14.75 1.8,15.72 6.62,20.55 6.62,24.26 2.08,28.8 2.08,43.62 1.36,44.35 1.36,47.51 3.11,49.26 8.23,49.26 9.47,50.5 R42.2 R27.1 9.69,49.06 9.21,49.06 8.5,48.35 8.5,46.77 7.4,45.67 7.4,42.36 7.18,42.14 Q4.1
SCK  (via drill 0.3, 0.3 pad 0.64)
  Top 0.203: U1.29 82.56,37.11 v82.56,35.87
  Top 0.305: R14.1 44.6,51.31 v45.11,50.8
  PWR 0.203: v82.56,35.87 82.56,36.54 83.18,37.16 88.08,37.16 89.66,38.74 89.66,47.56 87.25,49.97 v84.3,49.97
  Bottom 0.203: 82.76,49.61 83.94,49.61 v84.3,49.97
  Bottom 0.305: v45.11,50.8 45.18,50.73 70.68,50.73 71.38,50.03 82.34,50.03 82.76,49.61
SCL  (via drill 0.3)
  Top 0.203: 45.28,29.55 45.9,30.17 45.9,32.69 44.61,33.98 44.61,35.17 v45.56,36.12 | U1.7 85.82,46.9 85.21,47.51 78.56,47.51 77.64,48.43 v77.59,48.43 v77.59,48.42
  Top 0.305: L5.2 30.68,29.79 36.75,29.79 37.58,28.96 43.67,28.96 44.24,29.52 R58.1 45.28,29.55 46.64,29.55 SCL.TP
  PWR 0.203: v45.56,36.12 55.99,36.12 56.6,36.73 57.25,36.73 57.66,36.32 64.46,36.32 65.53,37.39 66.15,37.39 66.81,36.73 69.32,36.73 70.91,38.32 70.91,41.56 70.12,42.36 70.12,50.04 70.39,50.31 74.03,50.31 74.69,49.65 76.36,49.65 v77.59,48.42
SDA  (via drill 0.3)
  Top 0.203: R60.1 45.02,30.26 45.28,30.52 45.28,32.56 43.98,33.86 43.98,35.71 v44.89,36.62 | v78.52,48.9 78.52,48.87 79.43,47.95 85.36,47.95 86.22,47.09 U1.6
  Top 0.305: L6.2 30.97,35.49 30.97,31.01 31.4,30.58 38.16,30.58 39.17,29.57 42.1,29.57 42.35,29.82 R60.1 40.28,30.26 39.96,30.58 SDA.TP
  PWR 0.203: v44.89,36.62 45.4,37.13 56.43,37.13 64.63,37.13 65.34,37.84 69.65,37.84 70.4,38.59 70.4,41.2 69.51,42.09 69.51,50.31 70.12,50.92 76.5,50.92 v78.52,48.9
SEL  (via drill 0.3, 0.35)
  Top 0.203: v83.29,32.27 83.29,33.55 84.35,34.61 85.79,34.61 86.24,35.06 86.24,37.55 U1.37
  Top 0.305: v13.35,24.47 v13.34,24.47 K1.3
  GND 0.305: v39.3,31.59 38.12,30.41 19,30.41 16.79,28.2 16.25,28.2 v16.25,28.16
  PWR 0.305: v13.35,24.47 13.35,27.07 14.48,28.2 16.21,28.2 v16.25,28.16 | v39.3,31.59 39.47,31.43 80.65,31.43 81.49,32.27 v83.29,32.27
  Bottom 0.305: v13.35,24.47 13.35,23.33 12.08,22.06 SEL.TP
SS  (via drill 0.3, 0.3 pad 0.64)
  Top 0.203: v82.03,37.55 82.03,37.68 81.64,38.07 81.64,38.29 81.76,38.41 U1.28
  Top 0.305: R29.1 54.76,51.23 53.49,49.96 v53.49,48.53 v53.49,48.52
  PWR 0.203: v82.03,37.55 82.03,37.58 87.71,37.58 89.23,39.1 89.23,47.42 88.2,48.45 86.71,48.45 86.35,48.09 v86.35,47.92
  Bottom 0.305: v53.49,48.52 55.05,50.08 68.94,50.08 69.51,49.51 69.51,48.61 70.2,47.92 73.12,47.92 74.71,49.51 82.08,49.51 82.67,48.92 85.29,48.92 86.29,47.92 v86.35,47.92
SWCLK  (via drill 0.3)
  Top 0.203: U1.24 82.82,40.01 82.93,40.12 82.93,40.58 v83.44,41.09
  Bottom 0.203: JP1.4 89.15,41.23 88.26,42.12 87.48,42.12 87,41.64 84.17,41.64 83.62,41.09 v83.44,41.09
  Bottom 0.305: JP1.4 92.03,41.23 92.5,41.7 92.5,46.19 94.14,47.83 SWCLK.TP
SWDIO  (via drill 0.3)
  Top 0.203: v83.55,40.07 83.09,39.61 U1.25
  Bottom 0.203: v83.55,40.07 82.42,41.2 82.42,42.11 83.24,42.93 87.55,42.93 87.71,42.77 88.7,42.77 88.97,42.5 JP1.2
  Bottom 0.305: JP1.2 90.46,47.72 SWDIO.TP
USB_D+  (via drill 0.3, 0.35)
  Top 0.203: v15.83,4.32 v15.82,4.31 D4.2
  Top 0.305: USB_D+.2 20.52,27.45 v20.45,27.52
  PWR 0.305: v15.83,4.32 16.46,4.95 16.46,18.59 v17.37,19.5 17.5,19.63 17.5,26.98 18.04,27.52 v20.45,27.52
  Bottom 0.203: v15.83,4.32 16.45,4.94 J1.7 J1.6
  Bottom 0.305: USB-D+.TP 17.33,19.5 v17.37,19.5
USB_D-  (via drill 0.3, 0.35)
  Top 0.203: D4.1 v17.72,4.35 v17.71,4.35
  Top 0.305: USB_D-.2 20.48,25.64 v20.45,25.67
  PWR 0.305: v17.71,4.35 17.32,4.75 17.32,18.05 v18.78,19.5 18.18,20.1 18.18,24.45 19.47,25.74 20.38,25.74 v20.45,25.67
  Bottom 0.203: v17.71,4.35 17.45,4.62 J1.5 17.45,6.82 17.11,7.16 16.25,7.16 15.95,6.86 J1.8
  Bottom 0.305: USB-D-.TP 18.97,19.31 v18.78,19.5
USB_DM
  Top 0.203: U1.46 90.34,39.61 91.01,38.94 R63.2
USB_DP
  Top 0.203: U1.47 90.16,40.01 90.85,40.7 R38.2
VBUS_SENSE  (via drill 0.3, 0.35, 0.4)
  Top 0.203: U1.38 86.64,37.55 86.64,34.82 86.22,34.4 v86.22,34.18
  Top 0.305: D7.3 14.68,31.49 R50.1 13,31.51 C58.2 12.09,31.45 v11.73,31.8
  PWR 0.305: v11.73,31.8 13.19,33.26 32.77,33.26 34.94,35.44 57.78,35.44 58.18,35.83 65.4,35.83 65.8,36.23 v65.8,36.73
  Bottom 0.305: v65.8,36.73 67.51,38.44 72.28,38.44 74.4,36.32 76.33,36.32 78.65,34 86.04,34 v86.22,34.18 | v11.73,31.8 11.59,31.95 R51.2 11.59,38.51 VBUS_SENSE.TP
VCC  (via drill 0.3, 0.41 pad 0.9, 0.41 pad 0.91)
  Top 0.305: L7.1 47.3,33.47 49.44,31.32 D5.1 | U11.2 71,50.22
  Top 0.61: L7.1 46.38,33.5 v45.57,34.3 | U12.2 9.63,47.28 9.19,47.73 7.58,47.73 C18.1 | C18.1 | C18.1 v6.94,47.71
  Top 1.016: PTC1.1 8.09,33.81 v8.3,34.02 | v10.23,31.82 8.59,31.82 PTC1.1 | PTC1.1 8.09,29.31 8.67,28.73 v9.13,28.73 | v6.94,47.71 6.91,47.73 v6.05,47.73 5.96,47.83 C17.1 4.57,47.8 C21.1
  Bottom 0.305: C35.1 10.02,30.11 10.02,31.61 v10.23,31.82 | v6.05,47.73 5.34,47.73 5.31,47.72 | 5.31,47.72 5.27,47.67 C28.2 | R41.2 3.49,47.17 4.04,47.72 5.31,47.72
  other vias: 10.16,33.8 71.73,49.23 72.54,49.42 73.2,49.06 70.91,49.59 70.95,48.89 72.56,48.8
  pour Top: 7.52,34.55 11.09,34.55 11.12,34.51 11.12,27.9 7.52,27.9
  pour PWR (isolate 0.254, rank 2): 4.11,17.77 4.11,49.59 11.23,49.59 11.23,33.09 11.28,33.04 32.95,33.04 35.06,35.15 56.56,35.15 56.85,35.44 70.78,35.44 70.78,49.96 74.13,49.96 74.13,17.77
  pour Top: 70.61,50.71 72.8,50.71 73.15,50.36 76.97,50.36 77.01,50.32 77.01,48.83 76.76,48.58 70.6,48.58 70.6,50.69
VO_TPS  (via drill 0.3, 0.41 pad 0.91)
  Top 0.305: R12.1 34.32,39.76 v34.44,39.63 | 21.14,42.5 C19.2 | 22.75,42.48 C34.2 | v35.44,39.63 37.31,39.63 38,40.32 38,42.48 | C43.1 38,45.31 38,42.48 | U4.5 38.06,42.42 38,42.48
  Top 0.61: R11.2 21.14,42.5 | C19.2 22.75,42.48
  Top 0.813: C34.2 22.84,41.58 v23.01,41.41
  Bottom 0.305: C41.1 34.57,42.31 34.57,39.76 v34.44,39.63
  Bottom 0.813: 34.57,42.31 C39.1 C40.1 C42.1 25.64,42.25 23.85,42.25 v23.01,41.41 | C41.1 34.62,41.12
  other vias: 33.44,39.63 36.51,43.16 36.53,42.21 36.54,41.3 36.56,40.44 23.77,43.28 23.83,42.34
  pour Bottom: 22.25,43.56 22.25,40.77 31,40.77 32.57,39.2 36.81,39.2 36.81,43.56
  pour Top: 23.05,45.98 23.05,41.26 23.62,40.69 31.01,40.69 32.58,39.12 36.85,39.12 36.85,45.98
VOSEN  (via drill 0.3, 0.4)
  Top 0.203: U1.40 87.44,37.55 87.44,33.69 v87.75,33.38
  PWR 0.305: v20,29.04 21.2,30.24 34.66,30.24 36.69,32.27 38.22,32.27 38.78,32.83 39.94,32.83 40.28,32.48 65.83,32.48 66.17,32.82 v68.66,32.82 v68.67,32.81
  Bottom 0.305: R37.2 19.97,29.07 v20,29.04 20.77,29.81 D2.3 19.88,32.44 VOSEN.TP | v68.67,32.81 68.65,32.83 68.65,36.31 69.56,37.23 71.74,37.23 72.28,36.68 72.28,35.86 73.03,35.11 75.86,35.11 78.01,32.96 87.33,32.96 v87.75,33.38
  Bottom 0.61: R36.1 C13.2 R37.2
VOUT  (via drill 0.3 pad 0.64, 0.4 pad 0.64, 0.41 pad 0.91)
  Top 0.305: R12.2 34.32,35.95 | R1.2 38.37,37.04 35.42,37.04 v35.37,37.09
  Top 0.61: 34.32,35.95 v33.17,37.09 | K1.7 16.34,24.31 v16.06,24.6 15.34,23.88 K1.5
  Bottom 0.305: VOUT.TP 20.29,39.04 20.95,38.38
  Bottom 0.61: v33.17,37.09 33.03,37.09
  Bottom 0.813: D8.1 14.56,31.87 14.56,30 | v14.51,27.05 14.98,27.05 14.98,29.58 15.52,29.04 17.55,29.04 R37.1 | v14.51,27.05 14.55,27.01 14.55,26.15 | v14.51,27.05 14.36,26.9 14,26.9
  Bottom 1.016: 33.03,37.09 31.74,38.38 20.95,38.38 16.98,34.41 15.21,34.41 14.46,33.66 D8.1
  other vias: 15.46,25.5 15.66,27.05 34.27,37.09
  pour Top (isolate 0.254): 16.6,24.05 14.75,24.05 14.65,23.95 14.65,25.65 13.8,26.5 13.8,27.59 16.6,27.59
  pour Bottom (isolate 0.254, rank 2): 13.35,30.95 17.2,30.95 17.2,24.3 16.75,23.85 14.85,23.85 14.85,25.35 13.35,26.85
  pour Top (isolate 0.406, no thermals): 32.75,37.7 32.75,36.5 32.88,36.37 36.12,36.37 36.12,37.7
  pour Bottom (isolate 0.254, no thermals): 35.9,37.7 32.75,37.7 32.75,36.6 32.85,36.5 35.85,36.5 35.9,36.55
  pour Bottom: 31.96,38.63 36.18,38.63 36.34,38.47 36.34,34.04 36.09,33.79 32.44,33.79 32.07,34.16 32.07,37.46 31.6,37.93 31.6,38.27
XIN
  Top 0.203: U1.20 78.44,41.62
  Top 0.305: C59.2 X1.1 76.25,42.95 76.68,42.52 77.54,42.52 78.44,41.62
XOUT
  Top 0.203: U1.21 80.7,41.21 79.98,40.48 79.98,38.49 R46.1

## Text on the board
tPlace: MK2-RP2040 / v2-May-2023 | + | -
bPlace: VIN | GND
